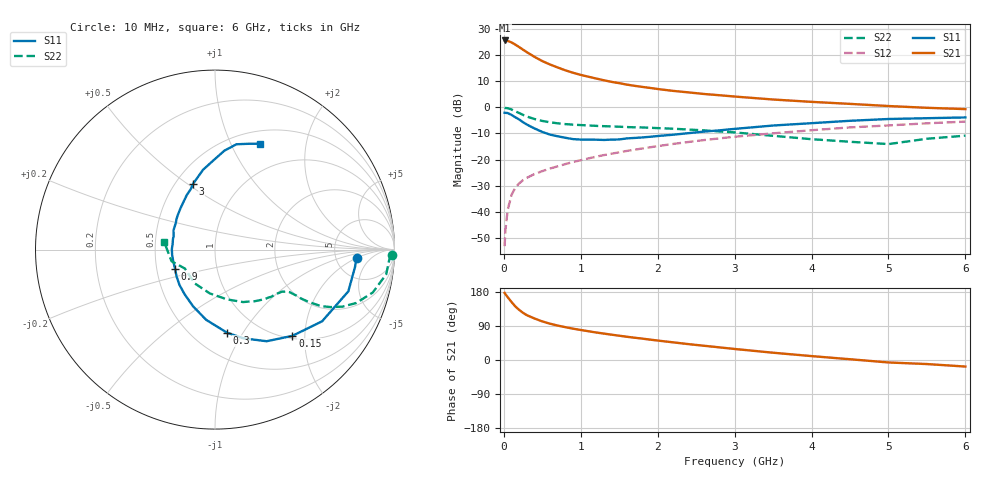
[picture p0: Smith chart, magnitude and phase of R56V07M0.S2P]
! SIEMENS Small Signal Semiconductors
! BFR183
! Si NPN RF Bipolar Junction Transistor in SOT23
! VCE = 6 V  IC = 7 mA
! Common Emitter S-Parameters:  May  1996
# GHz  S  MA  R  50
!  f  S11  S21  S12  S22
! GHz  MAG  ANG  MAG  ANG  MAG  ANG  MAG  ANG
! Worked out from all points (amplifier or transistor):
!   36 points, 10 MHz to 6 GHz, reference 50 ohm
!   highest |S21| = 25.6 dB at 10 MHz (marker M1)
!   |S21| within 3 dB of that: start of sweep to 222.6 MHz
!   unconditionally stable (mu >= 1): 923.2 MHz to 2.611 GHz
!   at 250 MHz: K = 0.50, MSG = 25.0 dB, |S12| = -27.9 dB
!   at 1.4 GHz: K = 1.06, MAG = 12.3 dB, |S12| = -17.7 dB
!   at 6 GHz: K = 0.88, MSG = 2.4 dB, |S12| = -5.5 dB
!   lowest NFmin = 1.25 dB at 450 MHz
!   S11 on the Smith chart (normalised r, x): 10 MHz: 8.03, -2.00; 150 MHz: 1.05, -1.73; 300 MHz: 0.72, -0.85; 900 MHz: 0.62, -0.14; 3 GHz: 0.61, +0.53; 6 GHz: 0.65, +1.30
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0.01  0.7903 -3.4  19.11 177.0  0.0022 93.2  0.9859 -1.6
0.02  0.7862 -7.0  19.1 173.9  0.0044 85.4  0.9726 -3.3
0.05  0.7784 -17.4  18.7 165.8  0.0109 81.0  0.9637 -8.2
0.1  0.7181 -33.8  17.55 153.0  0.0211 73.9  0.9111 -15.2
0.15  0.6456 -48.1  15.88 141.1  0.0292 67.7  0.8414 -20.7
0.2  0.586 -60.6  14.24 132.2  0.0351 64.8  0.7782 -24.1
0.25  0.5196 -72.1  12.71 124.4  0.0405 62.2  0.7178 -26.5
0.3  0.4682 -81.7  11.38 118.2  0.0449 60.7  0.6675 -28.1
0.4  0.3943 -97.2  9.247 109.4  0.053 59.7  0.5975 -29.2
0.5  0.3385 -111.2  7.689 101.8  0.0601 59.6  0.5504 -29.6
0.6  0.3013 -124.1  6.628 95.8  0.0675 60.2  0.5175 -29.5
0.7  0.2795 -135.0  5.801 90.9  0.0743 60.8  0.4953 -29.6
0.9  0.2468 -154.5  4.596 82.7  0.0901 61.5  0.4668 -30.0
1.1  0.2407 -172.7  3.859 75.9  0.1053 61.8  0.4504 -31.4
1.3  0.2378 173.0  3.303 69.7  0.1219 62.0  0.4366 -32.8
1.6  0.2548 155.3  2.727 61.3  0.1467 61.2  0.4197 -36.1
2.2  0.2993 130.1  2.068 46.6  0.1993 57.7  0.3905 -45.0
3  0.3874 108.2  1.612 29.1  0.2739 50.4  0.3318 -61.8
3.5  0.4492 98.6  1.414 19.2  0.3184 44.7  0.2854 -76.4
4.5  0.5534 84.6  1.166 2.0  0.4136 32.9  0.2195 -121.0
5.5  0.6204 71.9  0.981 -10.7  0.4952 21.0  0.2507 -165.0
6  0.6416 66.8  0.926 -17.3  0.5334 13.2  0.2874 171.0
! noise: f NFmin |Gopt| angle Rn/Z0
0.45  1.25  0.18  42  0.22
0.9  1.3  0.22  110  0.2
1.8  2  0.33  180  0.14
